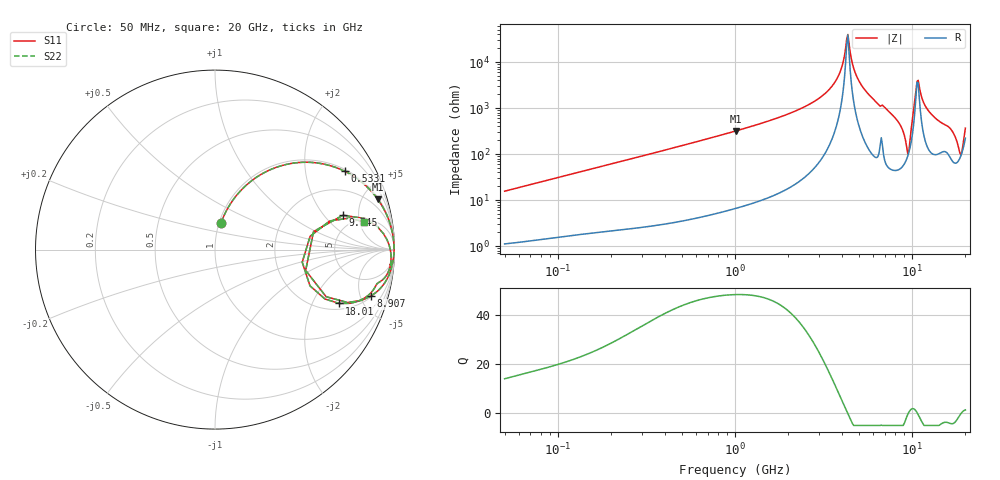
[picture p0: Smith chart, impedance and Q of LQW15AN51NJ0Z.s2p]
!Murata Part Number: LQW15AN51NJ0Z
!These Parameters are Measured in Series Mode Connection
!  o--[Z]--o
!Port1  Port2
!  o-------o
!Freq. Start=50[MHz] Stop=20[GHz], 401[Steps]
# Hz S RI R 50
!Freq.(Hz) S11(Real) S11(Imag) S21(Real) S21(Imag) S12(Real) S12(Imag) S22(Real) S22(Imag)
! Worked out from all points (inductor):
!   401 points, 50 MHz to 20 GHz, reference 50 ohm
!   read as one part in series: L = 49.6 nH near 51.52 MHz
!   highest Q = 48.2 at 1.015 GHz (marker M1), where L = 50.3 nH
!   self-resonance near 4.276 GHz
!   S11 on the Smith chart (normalised r, x): 50 MHz: 1.02, +0.31; 533.1 MHz: 1.07, +3.26; 8.907 GHz: 2.12, -6.08; 9.745 GHz: 3.82, +3.21; 18.01 GHz: 2.33, -3.25; 20 GHz: 5.45, +5.85
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5e7  0.0342 0.1493  0.9658 -0.1493  0.9658 -0.1493  0.0342 0.1493
1.364002e8  0.1598 0.3454  0.8402 -0.3454  0.8402 -0.3454  0.1598 0.3454
3.721004e8  0.5607 0.4837  0.4393 -0.4837  0.4393 -0.4837  0.5607 0.4837
5.330693e8  0.7222 0.4368  0.2778 -0.4368  0.2778 -0.4368  0.7222 0.4368
1e9  0.904 0.2844  0.096 -0.2844  0.096 -0.2844  0.904 0.2844
1.015091e9  0.9067 0.2807  0.0933 -0.2807  0.0933 -0.2807  0.9067 0.2807
2.728004e9  0.9917 0.0753  0.00829 -0.0753  0.00829 -0.0753  0.9917 0.0753
3.680849e9  0.9969 0.0264  0.00306 -0.0264  0.00306 -0.0264  0.9969 0.0264
4.34015e9  0.9976 -0.000544  0.00244 0.000544  0.00244 0.000544  0.9976 -0.000544
4.748272e9  0.9972 -0.0158  0.00283 0.0158  0.00283 0.0158  0.9972 -0.0158
5.117541e9  0.9964 -0.0292  0.00362 0.0292  0.00362 0.0292  0.9964 -0.0292
7.442007e9  0.9786 -0.118  0.0214 0.118  0.0214 0.118  0.9786 -0.118
8.907419e9  0.8664 -0.2602  0.1336 0.2602  0.1336 0.2602  0.8664 -0.2602
9.316812e9  0.6192 -0.2626  0.3808 0.2626  0.3808 0.2626  0.6192 -0.2626
9.745021e9  0.7124 0.1912  0.2876 -0.1912  0.2876 -0.1912  0.7124 0.1912
1.050288e10  0.9689 0.0286  0.0311 -0.0286  0.0311 -0.0286  0.9689 0.0286
1.082228e10  0.9786 -0.0117  0.0214 0.0117  0.0214 0.0117  0.9786 -0.0117
1.238412e10  0.9714 -0.1085  0.0286 0.1085  0.0286 0.1085  0.9714 -0.1085
1.646126e10  0.8814 -0.2255  0.1186 0.2255  0.1186 0.2255  0.8814 -0.2255
1.800918e10  0.6923 -0.3002  0.3077 0.3002  0.3077 0.3002  0.6923 -0.3002
1.88369e10  0.486 -0.0698  0.514 0.0698  0.514 0.0698  0.486 -0.0698
2e10  0.83 0.1543  0.17 -0.1543  0.17 -0.1543  0.83 0.1543
